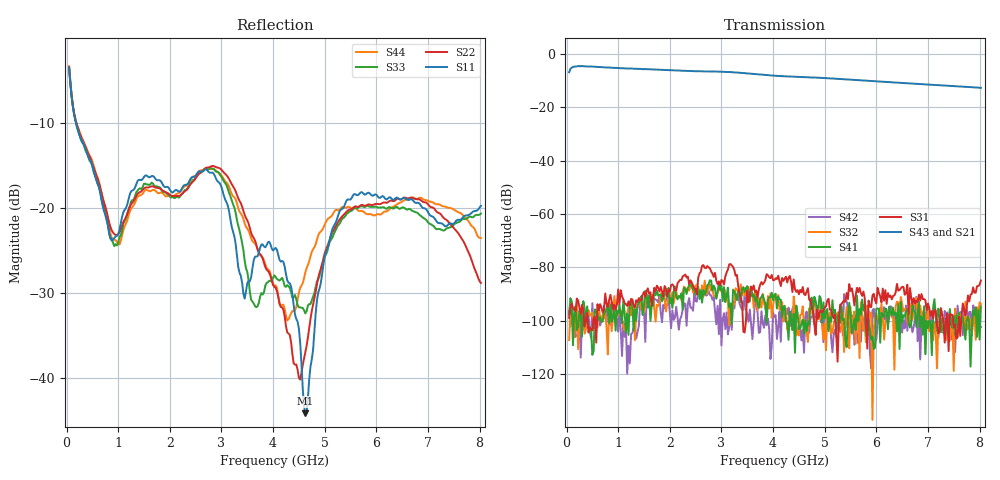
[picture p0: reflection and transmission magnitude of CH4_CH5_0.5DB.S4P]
!Agilent Technologies,E5071C,MY46316741,A.11.02
!Date: Mon Jun 01 11:48:37 2026
!Data & Calibration Information:
!1:CH4 INPUT 2:CH4 OUTPUT 3:CH5 INPUT 4:CH5 OUTPUT
!Freq	S11:SOLT4(ON)	S12:SOLT4(ON)	S13:SOLT4(ON)	S14:SOLT4(ON)
!	S21:SOLT4(ON)	S22:SOLT4(ON)	S23:SOLT4(ON)	S24:SOLT4(ON)
!	S31:SOLT4(ON)	S32:SOLT4(ON)	S33:SOLT4(ON)	S34:SOLT4(ON)
!	S41:SOLT4(ON)	S42:SOLT4(ON)	S43:SOLT4(ON)	S44:SOLT4(ON)
!PortZ  Port1:50+j0  Port2:50+j0  Port3:50+j0  Port4:50+j0
!Above PortZ is port z conversion or system Z0 setting when saving the data.
!When reading, reference impedance value at option line is always used.
# Hz S dB R 50
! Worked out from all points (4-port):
!   320 points, 50 MHz to 8.025 GHz, reference 50 ohm
!   strongest paths, dB at 50 MHz, 2.05 GHz, 4.05 GHz, 6.05 GHz, 8.025 GHz:
!     S43: -6.9, -6.2, -8.2, -10.3, -12.7
!     S21: -7.0, -6.3, -8.4, -10.6, -12.9
!     S31: -98.8, -86.3, -84.0, -89.5, -84.9
!     S41: -97.5, -95.1, -89.9, -95.6, -94.5
!     S32: -107.2, -89.2, -91.1, -99.1, -93.7
!     S42: -96.2, -96.1, -97.9, -97.8, -102.3
!   lowest |S11| = -44.2 dB at 4.625 GHz (marker M1), VSWR 1.01, Z = 50.6 + j0.102 ohm
!   |S11| at or under -10 dB: 183.1 MHz to end of sweep
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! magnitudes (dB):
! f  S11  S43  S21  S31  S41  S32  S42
! 50 MHz  -3.5  -6.9  -7.0  -98.8  -97.5  -107.2  -96.2
! 875 MHz  -23.9  -5.2  -5.3  -92.8  -100.3  -103.8  -93.1
! 2.85 GHz  -16.0  -6.6  -6.7  -83.5  -86.8  -90.6  -91.0
! 4.2 GHz  -26.4  -8.4  -8.6  -85.0  -94.7  -100.2  -97.0
! 4.625 GHz  -44.2  -8.7  -8.9  -90.4  -99.7  -100.4  -98.4
! 5.425 GHz  -19.2  -9.6  -9.8  -89.5  -109.8  -94.8  -92.6
! 8.025 GHz  -19.8  -12.7  -12.9  -84.9  -94.5  -93.7  -102.3
